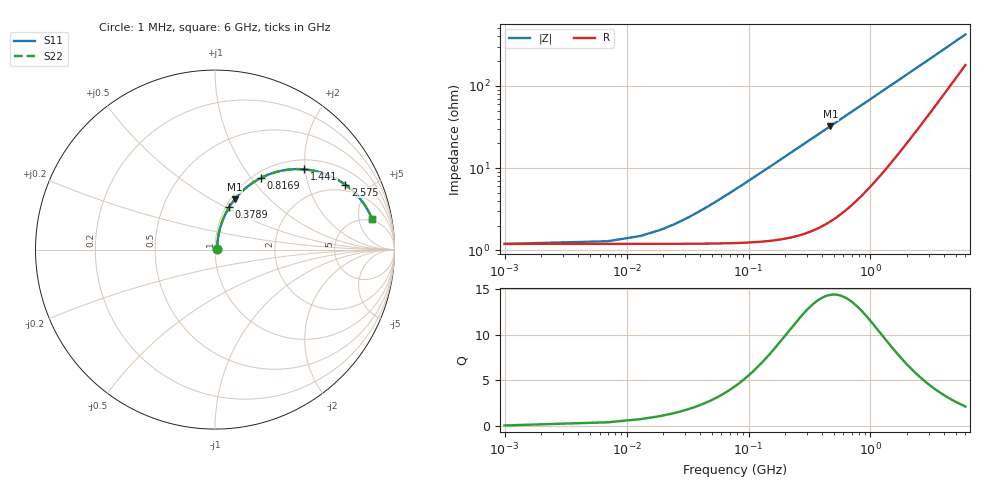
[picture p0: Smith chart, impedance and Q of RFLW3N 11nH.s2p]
!Vishay Electro-Films
!RFLW3N1100B - 11 nH Spiral Inductor on Quartz
!Measured in series configuration
!May 2011
# GHz S MA R 50
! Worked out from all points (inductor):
!   1001 points, 1 MHz to 6 GHz, reference 50 ohm
!   read as one part in series: L = 11 nH near 54.99 MHz
!   highest Q = 14.4 at 468.9 MHz (marker M1), where L = 11 nH
!   S11 on the Smith chart (normalised r, x): 1 MHz: 1.02, +0.00; 378.9 MHz: 1.04, +0.52; 816.9 MHz: 1.09, +1.13; 1.441 GHz: 1.22, +1.98; 2.575 GHz: 1.66, +3.51; 6 GHz: 4.58, +7.63
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0.001  0.01186 3.3  0.9882 -0.0  0.9882 -0.0  0.01186 3.3
0.018997  0.01755 46.8  0.9881 -0.7  0.9881 -0.7  0.01755 46.8
0.054991  0.0393 70.1  0.9873 -2.1  0.9873 -2.1  0.0393 70.1
0.072988  0.0511 73.5  0.9867 -2.8  0.9867 -2.8  0.0511 73.5
0.102983  0.07103 76.0  0.9852 -4.0  0.9852 -4.0  0.07103 76.0
0.132978  0.09103 76.9  0.9833 -5.2  0.9833 -5.2  0.09103 76.9
0.18097  0.1229 76.8  0.9792 -7.0  0.9792 -7.0  0.1229 76.8
0.234961  0.1583 75.8  0.9733 -9.1  0.9733 -9.1  0.1583 75.8
0.30095  0.2006 74.0  0.9641 -11.5  0.9641 -11.5  0.2006 74.0
0.378937  0.249 71.5  0.9508 -14.4  0.9508 -14.4  0.249 71.5
0.468922  0.3021 68.5  0.9325 -17.5  0.9325 -17.5  0.3021 68.5
0.624896  0.3865 63.3  0.8953 -22.7  0.8953 -22.7  0.3865 63.3
0.816864  0.4759 57.2  0.8433 -28.3  0.8433 -28.3  0.4759 57.2
1.00283  0.5477 52.0  0.7906 -33.1  0.7906 -33.1  0.5477 52.0
1.44076  0.6693 41.9  0.672 -41.7  0.672 -41.7  0.6693 41.9
1.71671  0.7205 37.0  0.6068 -45.6  0.6068 -45.6  0.7205 37.0
2.00467  0.7599 32.8  0.5477 -48.7  0.5477 -48.7  0.7599 32.8
2.57457  0.8107 26.5  0.4543 -52.8  0.4543 -52.8  0.8107 26.5
3.0005  0.8345 23.0  0.4006 -54.6  0.4006 -54.6  0.8345 23.0
4.00233  0.8666 17.3  0.3107 -56.2  0.3107 -56.2  0.8666 17.3
5.00417  0.8827 13.6  0.2521 -55.7  0.2521 -55.7  0.8827 13.6
6  0.8917 11.0  0.2115 -53.8  0.2115 -53.8  0.8917 11.0
